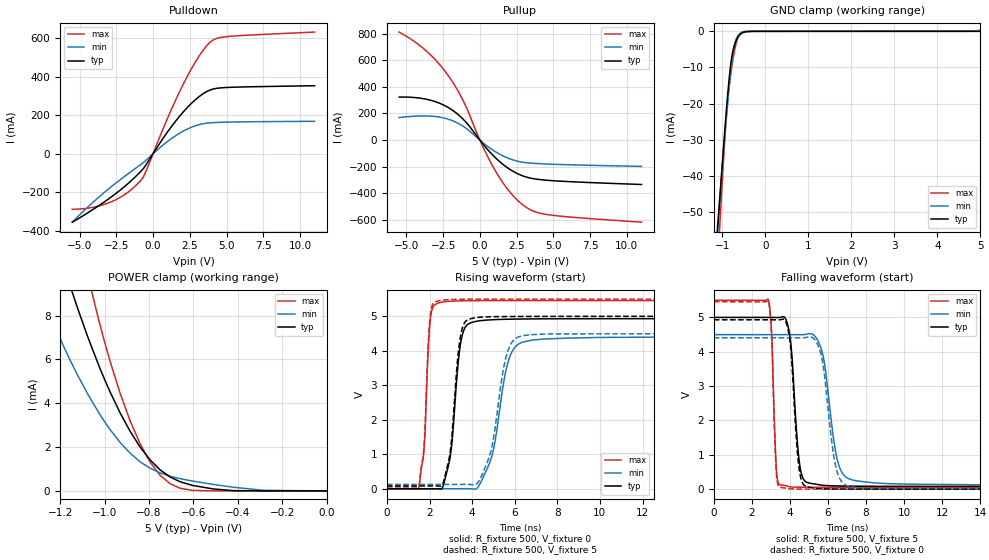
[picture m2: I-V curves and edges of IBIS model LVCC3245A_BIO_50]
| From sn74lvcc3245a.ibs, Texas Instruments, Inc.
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[Model]   LVCC3245A_BIO_50
Model_type  I/O
Vinl=1.65
Vinh=3.85
Enable   Active-Low
Vref =   0
Rref =   500
Cref =   50p
Vmeas =   2.5
| variable   typ   min   max
C_comp   18.50pF   NA   NA
| C_pullup   14.39pF   8.23pF   22.24pF
| C_pulldown   7.63pF   5.05pF   10.24pF
| C_tri-state   7.35pF   6.31pF   8.54pF
[Temperature Range]   40   100   -40
| Ambient temperature   25   85   -40
[Voltage range]   5   4.5   5.5
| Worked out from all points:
|   slope of the pulldown table from 0 to 0.75 V, typ, clamps not added: 8.6 ohm
|   slope of the pullup table from 0 to 0.75 V, typ, clamps not added: 7.64 ohm
|   GND clamp passes 1 mA (typ) near -0.60 V on its own axis
|   POWER clamp passes 1 mA (typ) near -0.75 V on its own axis
|   rising waveform, R_fixture 500, V_fixture 0: 20-80 % time 414ps typ, 730ps min, 233ps max; typ from 0 V to 4.93 V
|   falling waveform, R_fixture 500, V_fixture 5: 20-80 % time 355ps typ, 610ps min, 189ps max; typ from 5 V to 0.081 V
|   rising waveform, R_fixture 500, V_fixture 5: 20-80 % time 395ps typ, 679ps min, 228ps max; typ from 0.081 V to 5 V
|   falling waveform, R_fixture 500, V_fixture 0: 20-80 % time 341ps typ, 564ps min, 186ps max; typ from 4.93 V to 0 V
[GND Clamp]
| LVCC3245A_BIO_50
|   Voltage   I(typ)   I(min)   I(max)
-5.5V     -941.9mA   -838.1mA   -1.112A
-1.14V    -60.07mA   -57.95mA   -71.26mA
-1.09V    -51.46mA   -50.37mA   -60.23mA
-1.05V    -44.67mA   -44.38mA   -51.55mA
-910mV    -22.27mA   -24.34mA   -23.99mA
-860mV    -15.31mA   -17.8mA    -17.14mA
-805mV    -9.103mA   -11.34mA   -11.86mA
-750mV    -5.157mA   -6.125mA   -7.557mA
-695mV    -3.004mA   -2.768mA   -4.107mA
-620mV    -1.327mA   -933.2uA   -1.209mA
-550mV    -517.7uA   -425.5uA   -250.5uA
5V        2.452nA    280.9uA    47.45pA
[POWER Clamp]
| LVCC3245A_BIO_50
|   Voltage   I(typ)   I(min)   I(max)
-5.5V     376.1mA    259.6mA    632.7mA
-1.285V   13.82mA    8.979mA    20.69mA
-1.155V   9.363mA    5.967mA    13.54mA
-1.125V   8.444mA    5.355mA    12.07mA
-1.075V   7.01mA     4.405mA    9.803mA
-1.025V   5.697mA    3.55mA     7.745mA
-975mV    4.512mA    2.796mA    5.908mA
-840mV    2.001mA    1.33mA     2.143mA
-795mV    1.414mA    1.035mA    1.314mA
-705mV    634.9uA    672.5uA    329.3uA
-510mV    88.78uA    296.1uA    1.009uA
-95.1fV   2.452nA    11.28nA    58.09pA
[Pulldown]
| LVCC3245A_BIO_50
|   Voltage   I(typ)   I(min)   I(max)
-5.5V     -355.3mA   -354.7mA   -288.4mA
-4.095V   -289.8mA   -252.7mA   -278.2mA
-2.83V    -223.5mA   -170.3mA   -249mA
-1.755V   -158.2mA   -107.2mA   -202.5mA
-800mV    -89.07mA   -54.27mA   -135.5mA
-500mV    -59.78mA   -35.05mA   -93.78mA
995mV     113.8mA    64.1mA     185.5mA
2.115V    221.6mA    119.5mA    369.4mA
3.17V     297.9mA    151.4mA    510.7mA
3.985V    332.9mA    160.6mA    584.1mA
5.21V     344mA      164mA      608.4mA
11V       352.5mA    167.9mA    630.6mA
[Pullup]
| LVCC3245A_BIO_50
|   Voltage   I(typ)   I(min)   I(max)
-5.5V     323mA      169.2mA    811.5mA
-3.675V   307.6mA    181.6mA    672.3mA
-2.88V    282.7mA    174.8mA    585.1mA
-2.165V   245.4mA    157.2mA    486.4mA
-1.13V    155.8mA    103.1mA    294.2mA
135mV     -19.18mA   -12.9mA    -33.13mA
1.005V    -127mA     -83.84mA   -221.6mA
1.95V     -213.3mA   -137.1mA   -377.8mA
2.9V      -268.2mA   -166.1mA   -484.9mA
3.665V    -290.3mA   -174.8mA   -535mA
4.6V      -302mA     -180mA     -559.9mA
11V       -333.5mA   -197.5mA   -616.9mA
[Ramp]
| LVCC3245A_BIO_50
| variable   typ   min   max
dV/dt_r   2.97/4.24E-10   2.65/7.36E-10   3.28/2.35E-10
dV/dt_f   2.96/3.66E-10   2.64/6.14E-10   3.29/1.93E-10
R_load = 500
[Rising Waveform]
| LVCC3245A_BIO_50
R_fixture =   500
C_fixture =   0
L_fixture =   0
V_fixture =   0
V_fixture_min = 0
V_fixture_max = 0
|   Time   V(typ)   V(min)   V(max)
0s        259.1pV    88.49nV    136.8pV
1.495ns   -265.7nV   144.5nV    21.6mV
1.755ns   -8.339uV   256.2nV    1.278V
2.03ns    -39.21uV   -266.7nV   4.879V
2.415ns   -114.2uV   7.844uV    5.385V
2.97ns    933.4mV    -48.83uV   5.437V
3.49ns    4.329V     777.1uV    5.449V
3.935ns   4.813V     -1.611mV   5.453V
6.375ns   4.922V     4.252V     5.456V
24.99ns   4.931V     4.408V     5.456V
[Falling Waveform]
| LVCC3245A_BIO_50
R_fixture =   500
C_fixture =   0
L_fixture =   0
V_fixture =   5
V_fixture_min = 4.5
V_fixture_max = 5.5
|   Time   V(typ)   V(min)   V(max)
0s        5V         4.5V       5.5V
2.88ns    5V         4.5V       5.509V
3.29ns    4.999V     4.5V       601.8mV
3.485ns   5.001V     4.5V       128.3mV
3.99ns    4.5V       4.5V       68.99mV
4.48ns    870mV      4.498V     57.5mV
4.895ns   198.2mV    4.514V     56.95mV
5.655ns   119.2mV    4.078V     56.2mV
7.145ns   88.51mV    292.5mV    55.91mV
24.99ns   81.21mV    125.3mV    55.88mV
[Rising Waveform]
| LVCC3245A_BIO_50
R_fixture =   500
C_fixture =   0
L_fixture =   0
V_fixture =   5
V_fixture_min = 4.5
V_fixture_max = 5.5
|   Time   V(typ)   V(min)   V(max)
0s        81.21mV    125.3mV    55.88mV
1.495ns   81.21mV    125.3mV    77.04mV
1.745ns   81.2mV     125.3mV    1.284V
2.015ns   81.17mV    125.3mV    4.923V
2.325ns   83.02mV    125.3mV    5.434V
2.92ns    887.3mV    125.3mV    5.485V
3.41ns    4.256V     125.6mV    5.494V
3.855ns   4.92V      126.3mV    5.497V
6.2ns     4.995V     4.408V     5.5V
24.99ns   5V         4.5V       5.5V
[Falling Waveform]
| LVCC3245A_BIO_50
R_fixture =   500
C_fixture =   0
L_fixture =   0
V_fixture =   0
V_fixture_min = 0
V_fixture_max = 0
|   Time   V(typ)   V(min)   V(max)
0s        4.931V     4.408V     5.456V
2.88ns    4.931V     4.408V     5.463V
3.28ns    4.93V      4.408V     552.5mV
3.485ns   4.932V     4.408V     57.99mV
3.965ns   4.47V      4.408V     13.04mV
4.455ns   741.8mV    4.407V     4.247mV
4.875ns   74.83mV    4.42V      2.784mV
5.625ns   15mV       3.954V     947uV
7.01ns    2.882mV    100.3mV    125.6uV
24.99ns   661.2nV    3.224uV    266.9nV
